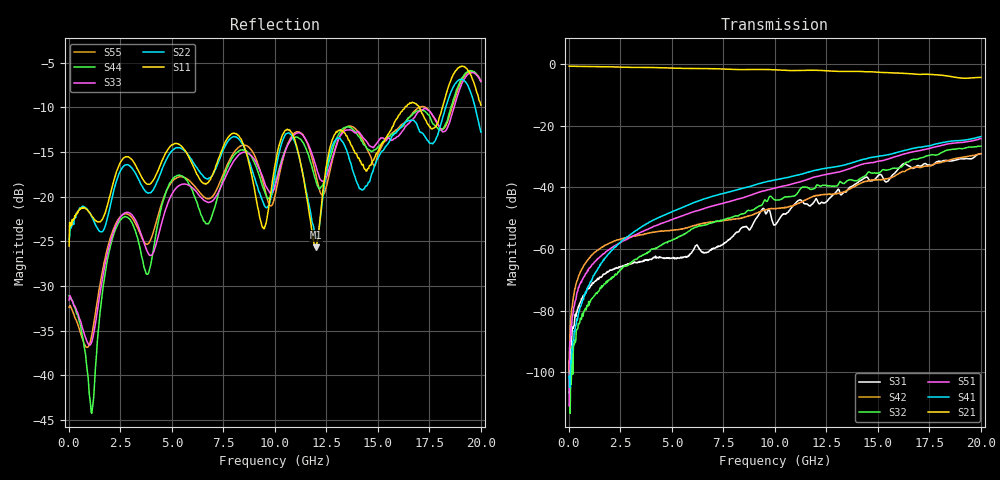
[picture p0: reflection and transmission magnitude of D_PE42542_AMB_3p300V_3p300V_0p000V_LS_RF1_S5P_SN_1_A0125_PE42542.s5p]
! Device ID: PE42542
! Device ID: PE42542
! File Path: z:\PE42542\PE42543_20140723_inv\AMB\3p300\LS_RF1\PE42542_AMB_3p300V_3p300V_0p000V_LS_RF1_S5P_SN_1_A0125_PE42542.s5p
! Serial: 1
! Lot: A0125_PE42542
! Temp: AMB
! VDD: 3.300
! VSS: 0.000
! Control_Hi: 3.300
! Control_Lo: 0.000
! Logic State: LS_RF1
! Port 1: RFC
! Port 2: RF1
! Port 3: RF2
! Port 5: RF3
! Port 6: RF4
! ThroughPath:1-2
! IDD: -0.000143858362
! ISS: -1.77882305e-010
#  Hz  S  RI  R  50
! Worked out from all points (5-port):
!   801 points, 10 MHz to 20 GHz, reference 50 ohm
!   strongest paths, dB at 10 MHz, 5.008 GHz, 10.01 GHz, 15 GHz, 20 GHz:
!     S21: -0.7, -1.3, -1.9, -2.6, -4.3
!     S41: -101.2, -47.9, -37.6, -30.0, -23.5
!     S51: -110.8, -50.4, -40.2, -31.5, -24.2
!     S32: -106.3, -57.1, -44.0, -35.3, -26.6
!     S42: -99.6, -53.9, -46.9, -37.5, -29.0
!     S31: -96.4, -62.9, -52.1, -36.3, -29.1
!   lowest |S11| = -25.7 dB at 11.98 GHz (marker M1), VSWR 1.11, Z = 51.4 + j5.08 ohm
!   |S11| at or under -10 dB: start of sweep to 16.32 GHz; 17.01 GHz to 18.14 GHz (1.129 GHz wide, 6.43 % of centre)
